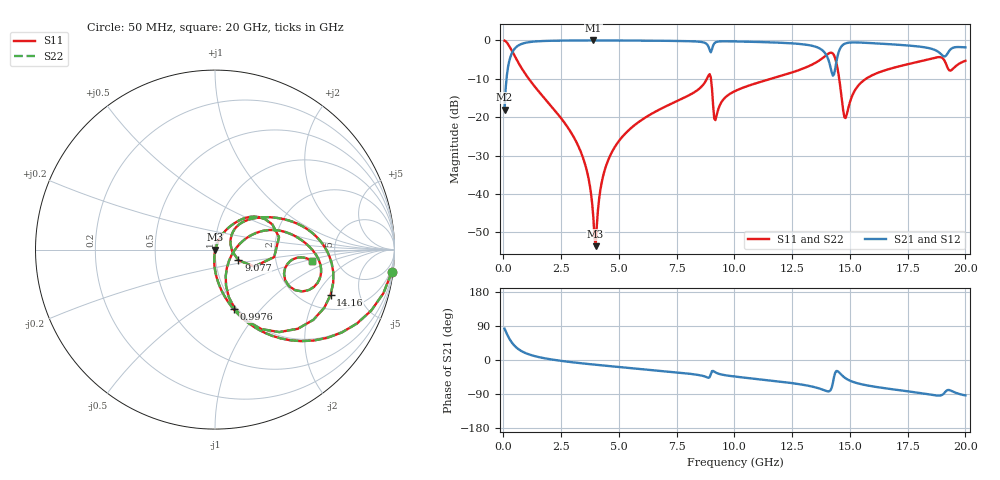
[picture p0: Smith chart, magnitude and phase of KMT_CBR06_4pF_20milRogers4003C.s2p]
! Data measured by Modelithics Inc. support@modelithics.com 813-866-6335
! KEMET CBR0603 4pF, Pad Width= 0.851mm, Pad Length= 0.64mm, Pad Gap= 0.62mm, 20mil Rogers 4003C substrate Data, January 2022
# hz S ma R 50
! 2 Port Network Data from SP1.SP block
! freq  magS11  angS11  magS21  angS21  magS12  angS12  magS22  angS22
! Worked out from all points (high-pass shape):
!   401 points, 50 MHz to 20 GHz, reference 50 ohm
!   highest |S21| = -0.02 dB at 3.89 GHz (marker M1); lowest = -18.0 dB at 50 MHz (marker M2)
!   |S21| within 3 dB of the highest: 391.7 MHz to 8.97 GHz (8.578 GHz wide, 183 % of centre); 8.984 GHz to 13.88 GHz (4.899 GHz wide, 42.8 % of centre)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
!   lowest |S11| = -53.6 dB at 3.99 GHz (marker M3), VSWR 1.00, Z = 50.2 + j0.018 ohm
!   |S11| at or under -10 dB: 1.097 GHz to 8.807 GHz (7.711 GHz wide, 156 % of centre); 8.985 GHz to 11.58 GHz (2.599 GHz wide, 25.3 % of centre); 14.54 GHz to 15.7 GHz (1.161 GHz wide, 7.68 % of centre)
!   |S22| runs from -53.6 to -0.1 dB; largest |S21 - S12| = 0
!   S11 on the Smith chart (normalised r, x): 50 MHz: 1, -15; 997.6 MHz: 0.96, -0.73; 9.077 GHz: 1.29, -0.16; 14.16 GHz: 2.74, -2.65; 20 GHz: 3.26, -0.58
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5e7  0.992 -7.4  0.1257 82.6  0.1257 82.6  0.992 -7.4
3.4925e8  0.7461 -42.8  0.665 47.2  0.665 47.2  0.7461 -42.8
9.97625e8  0.3481 -72.6  0.9363 17.2  0.9363 17.2  0.3481 -72.6
3.391625e9  0.03277 -95.5  0.9975 -8.7  0.9975 -8.7  0.03277 -95.5
3.690875e9  0.01554 -93.6  0.9978 -10.7  0.9978 -10.7  0.01554 -93.6
3.890375e9  0.005007 -78.8  0.9979 -11.9  0.9979 -11.9  0.005007 -78.8
3.990125e9  0.00209 4.9  0.9979 -12.5  0.9979 -12.5  0.00209 4.9
4.289375e9  0.01585 68.2  0.9977 -14.3  0.9977 -14.3  0.01585 68.2
4.73825e9  0.03711 69.7  0.997 -16.9  0.997 -16.9  0.03711 69.7
6.73325e9  0.1248 60.5  0.9891 -28.2  0.9891 -28.2  0.1248 60.5
8.877875e9  0.3491 23.8  0.8277 -46.8  0.8277 -46.8  0.3491 23.8
9.077375e9  0.1432 -24.4  0.8568 -28.8  0.8568 -28.8  0.1432 -24.4
9.227e9  0.1048 33.7  0.9555 -34.2  0.9555 -34.2  0.1048 33.7
1.0025e10  0.2188 44.6  0.969 -43.7  0.969 -43.7  0.2188 44.6
1.336662e10  0.4847 17.1  0.8505 -70.1  0.8505 -70.1  0.4847 17.1
1.416462e10  0.6917 -21.4  0.4435 -79.5  0.4435 -79.5  0.6917 -21.4
1.4414e10  0.5113 -59.9  0.5255 -29.0  0.5255 -29.0  0.5113 -59.9
1.4813e10  0.09745 -18.1  0.914 -48.2  0.914 -48.2  0.09745 -18.1
1.546138e10  0.2777 21.6  0.9363 -63.4  0.9363 -63.4  0.2777 21.6
1.670825e10  0.4245 12.2  0.8927 -76.2  0.8927 -76.2  0.4245 12.2
1.910225e10  0.54 -25.6  0.6163 -86.1  0.6163 -86.1  0.54 -25.6
2e10  0.5424 -6.6  0.8102 -93.5  0.8102 -93.5  0.5424 -6.6
